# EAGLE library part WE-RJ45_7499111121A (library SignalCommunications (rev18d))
RJ45 LAN Transformer Characteristics RJ45 connector with integrated transformer common mode choke Available in SMD, THT and THT with USB 350 μH min. OCL with 8 mA bias Complies with IEEE 802.3 Extended temperature range from –40 °C to +85 °C available PoE/PoE+ Applications XDSL Modems Embedded PC LAN network applications Hub, Router, Switches Details see: http://katalog.we-online.de/en/pbs/WE-LAN_RJ45/7499010441? Updated by Yingchun Shan 2016-08-29 2016(C) Würth Elektronik
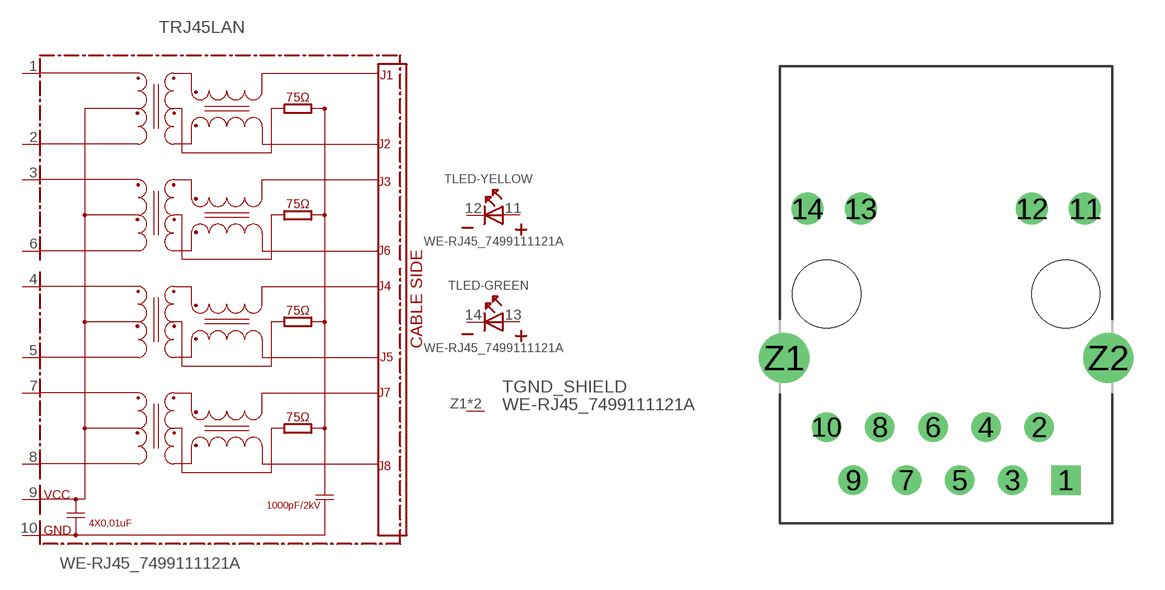
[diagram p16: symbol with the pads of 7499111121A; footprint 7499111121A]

Designator prefix T; gates RJ45LAN=7499111121A LED-YELLOW=LED2PIN LED-GREEN=LED2PIN GND_SHIELD=GNDPIN

## WE-RJ45_7499111121A (COMPANY-URL: http://www.we-online.de; CREATED-BY: Christin Zierenner; CREATED-DATE: AUG 2012; DATASHEET-URL: http://katalog.we-online.de/kataloge/eisos/media/pdf/7499111121A.pdf; MANUFACTURER: Würth Elektronik eiSos GmbH)  [7499111121A]
1  RJ45LAN:1
2  RJ45LAN:2
3  RJ45LAN:3
4  RJ45LAN:4
5  RJ45LAN:5
6  RJ45LAN:6
7  RJ45LAN:7
8  RJ45LAN:8
9  RJ45LAN:9  pwr
10  RJ45LAN:10  pwr
11  LED-YELLOW:A  pas
12  LED-YELLOW:K  pas
13  LED-GREEN:A  pas
14  LED-GREEN:K  pas
Z1  GND_SHIELD:GND  pwr
Z2  GND_SHIELD:GND  pwr

## Footprint 7499111121A (pad centres in mm)
MAX HEIGHT=13.95mm PORTS----1X1 LED --YES
drill 0.9 square: 1 5.715,-8.89
drill 0.9: 2 4.445,-6.35; 3 3.175,-8.89; 4 1.905,-6.35; 5 0.635,-8.89; 6 -0.635,-6.35; 7 -1.905,-8.89; 8 -3.175,-6.35; 9 -4.445,-8.89; 10 -5.715,-6.35
drill 1.02: 11 6.63,4.08; 12 4.09,4.08; 13 -4.09,4.08; 14 -6.63,4.08
drill 1.6: Z1 -7.745,-3.05; Z2 7.745,-3.05
hole 3.25 at 5.715,0
hole 3.25 at -5.715,0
